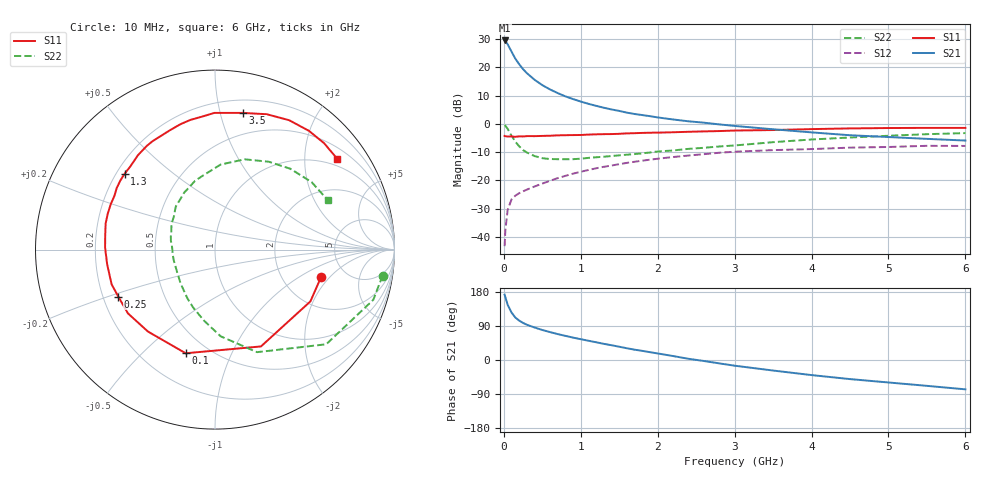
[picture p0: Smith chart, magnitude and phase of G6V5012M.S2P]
! SIEMENS Small Signal Semiconductors
! BFG193
! Si NPN RF Bipolar Junction Transistor in SOT223
! VCE = 0.5 V  IC = 12 mA
! Common Emitter S-Parameters:  August  1996
# GHz  S  MA  R  50
!  f  S11  S21  S12  S22
! GHz  MAG  ANG  MAG  ANG  MAG  ANG  MAG  ANG
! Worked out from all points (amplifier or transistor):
!   36 points, 10 MHz to 6 GHz, reference 50 ohm
!   highest |S21| = 29.5 dB at 10 MHz (marker M1)
!   |S21| within 3 dB of that: start of sweep to 81.63 MHz
!   unconditionally stable (mu >= 1): 712.9 MHz to 4.954 GHz; 5.649 GHz to end of sweep
!   at 250 MHz: K = 0.63, MSG = 21.6 dB, |S12| = -23.8 dB
!   at 1.4 GHz: K = 1.11, MAG = 7.9 dB, |S12| = -14.7 dB
!   at 6 GHz: K = 1.01, MAG = 0.4 dB, |S12| = -7.8 dB
!   S11 on the Smith chart (normalised r, x): 10 MHz: 3.29, -1.60; 100 MHz: 0.38, -0.68; 250 MHz: 0.26, -0.21; 1.3 GHz: 0.23, +0.35; 3.5 GHz: 0.31, +1.18; 6 GHz: 0.79, +2.84
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0.01  0.6105 -14.5  29.75 172.3  0.0069 85.5  0.945 -8.8
0.02  0.6048 -28.5  29.02 165.6  0.0134 79.6  0.9254 -17.6
0.05  0.5972 -64.6  25.39 145.5  0.0304 63.1  0.8138 -40.4
0.1  0.6002 -105.8  18.89 125.2  0.0463 50.0  0.6176 -67.7
0.15  0.59 -129.3  14.14 112.0  0.0539 44.2  0.4839 -86.3
0.2  0.6013 -143.8  11.29 103.9  0.0596 42.6  0.3999 -98.9
0.25  0.599 -154.1  9.257 97.8  0.0643 41.9  0.3442 -110.9
0.3  0.6076 -161.4  7.852 93.0  0.0689 42.6  0.3116 -119.6
0.4  0.6064 -172.2  6.002 85.7  0.0783 43.7  0.2693 -135.3
0.5  0.6123 179.1  4.829 79.2  0.088 44.1  0.2476 -147.5
0.6  0.6168 172.7  4.058 73.7  0.0987 45.1  0.2392 -157.0
0.7  0.6263 166.6  3.497 68.4  0.1099 45.1  0.2373 -165.6
0.8  0.6302 161.5  3.059 63.7  0.1205 44.5  0.2372 -173.3
1.1  0.646 148.0  2.258 50.8  0.1532 41.6  0.2505 168.8
1.3  0.6577 139.9  1.926 42.6  0.1744 38.5  0.2624 158.2
1.7  0.6841 126.4  1.493 27.2  0.214 31.0  0.2925 141.9
2.2  0.7101 111.0  1.195 10.4  0.2594 19.8  0.3386 125.4
2.8  0.7458 95.0  0.978 -8.9  0.3086 6.3  0.3983 106.4
3.5  0.7772 78.5  0.802 -27.8  0.3433 -10.8  0.4745 86.3
4.5  0.8308 60.2  0.629 -50.4  0.3801 -29.4  0.5737 58.6
5.5  0.8491 44.3  0.543 -68.2  0.4092 -50.9  0.6568 34.9
6  0.8484 36.5  0.507 -77.4  0.4073 -63.2  0.6867 23.5
